{attribute 'qualified_only'}
VAR_GLOBAL
//************************HW-IO******************************************
	NDI									:STR_NDI;	
	NDO									:STR_NDO;
	AI									:STR_AI;
	AO									:STR_AO;	
	//POWER
	TURBO_PUMP_POWER_ON 				:BOOL;
	PENDULUM_VALVE_HEATER_POWER_ON		:BOOL;
	LID_HEATER_POWER_ON					:BOOL;
	CHAMBER_HEATER_POWER_ON				:BOOL;
	IGS_HEATER_POWER_ON					:BOOL;
	TAPE_HEATER_POWER_ON				:BOOL;
	FORELINE_HEATER_POWER_ON			:BOOL;
	GATE_VALVE_HEATER_POWER_ON			:BOOL;	
	//HEATER	
	LID_HEATER_AUTO_TUNE_EN				:ARRAY[1..10] OF BOOL;
	CHAMBER_HEATER_AUTO_TUNE_EN			:ARRAY[1..10] OF BOOL;
	PEN_VALVE_HEATER_AUTO_TUNE_EN		:BOOL;
	GATE_VALVE_HEATER_AUTO_TUNE_EN		:BOOL;
	IGS_HEATER_AUTO_TUNE_EN				:ARRAY[1..10] OF BOOL;
	TAPE_HEATER_AUTO_TUNE_EN			:ARRAY[1..10] OF BOOL;
	FORELINE_HEATER_AUTO_TUNE_EN		:ARRAY[1..20] OF BOOL;
	STAGE_HEATER_AUTO_TUNE_EN			:ARRAY[1..10] OF BOOL;
	
	LID_HEATER_AUTO_TUNE_OUTPUT			:ARRAY[1..10] OF REAL;
	CHAMBER_HEATER_AUTO_TUNE_OUTPUT		:ARRAY[1..10] OF REAL;
	PEN_VALVE_HEATER_AUTO_TUNE_OUTPUT	:REAL;
	GATE_VALVE_HEATER_AUTO_TUNE_OUTPUT	:REAL;
	IGS_HEATER_AUTO_TUNE_OUTPUT			:ARRAY[1..10] OF REAL;
	TAPE_HEATER_AUTO_TUNE_OUTPUT		:ARRAY[1..10] OF REAL;
	FORELINE_HEATER_AUTO_TUNE_OUTPUT	:ARRAY[1..20] OF REAL;
	STAGE_HEATER_AUTO_TUNE_OUTPUT		:ARRAY[1..10] OF REAL;
	
	LID_HEATER_SSR_ON					:ARRAY[1..10] OF BOOL;
	CHAMBER_HEATER_SSR_ON				:ARRAY[1..10] OF BOOL;
	PEN_VALVE_HEATER_SSR_ON				:BOOL;
	GATE_VALVE_SSR_ON					:BOOL;
	IGS_HEATER_SSR_ON					:ARRAY[1..10] OF BOOL;
	TAPE_HEATER_SSR_ON					:ARRAY[1..10] OF BOOL;
	FORELINE_HEATER_SSR_ON				:ARRAY[1..20] OF BOOL;
	STAGE_HEATER_SCR_OUTPUT				:ARRAY[1..10] OF REAL;	
//INTERLOCK
	ALARM_OCC				:BOOL;
	WARNING_OCC				:BOOL;	
//UI-Config
	PMConfig				:ConfigPM;	
	Chiller					:ConfigChiller;	
	InnerChiller			:ConfigChiller;
	OuterChiller			:ConfigChiller;
	TopChiller				:ConfigChiller;
	DryPump					:ConfigDryPump;	
	Mfcgas1					:ConfigMfcGas;
	MfcN2					:ConfigMfcGas;
	MfcHe					:ConfigMfcGas; 	
	Pump					:ConfigPump;	
	Purge					:ConfigPurge;	
	PendulumHeater			:ConfigHeater;
	LidHeater				:ConfigHeater;
	ChamberHeater			:ConfigHeater;
	ForelineHeater			:ConfigHeater;
	STAGE					:ConfigHeater;
	PendulumValve			:ConfigPendulumValve;	
//UI-RECIPE
	Process_Start			:BOOL;
	Process_Stop			:BOOL;
	Step_Num				:INT;
	SetpArray				:ARRAY[1..100] OF RecipeEachStep;	
//INTERLOCK
	TurboN2PurgePressure	:INT;	//PS103	
END_VAR
